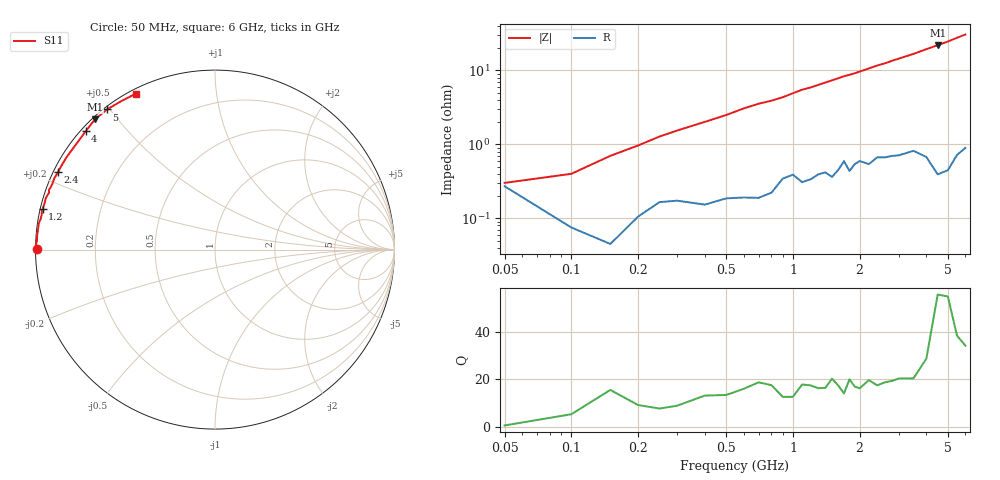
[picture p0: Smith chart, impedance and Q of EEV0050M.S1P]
! Infineon Technologies  Discrete & RF Semiconductors
! BBY55-02W
! Si Tuning Diode in SCD-80
! VR =
! S-Parameters:  June  2000
# GHz  S  MA  R  50
!  f  S11
! GHz  MAG  ANG
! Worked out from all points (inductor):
!   34 points, 50 MHz to 6 GHz, reference 50 ohm
!   read as one part to ground: L = 741 pH near 100 MHz
!   highest Q = 55 at 4.5 GHz (marker M1), where L = 776 pH
!   S11 on the Smith chart (normalised r, x): 50 MHz: 0.01, +0.00; 1.2 GHz: 0.01, +0.12; 2.4 GHz: 0.01, +0.23; 4 GHz: 0.01, +0.39; 5 GHz: 0.01, +0.49; 6 GHz: 0.02, +0.61
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0.05  0.9892 179.7
0.1  0.997 179.1
0.15  0.9982 178.4
0.25  0.9934 177.1
0.5  0.9926 174.3
0.6  0.9924 173.0
0.7  0.9925 171.9
0.8  0.9912 171.1
0.9  0.9864 170.1
1  0.9847 168.8
1.1  0.9879 167.5
1.2  0.9868 166.6
1.4  0.9837 164.4
1.5  0.9859 163.3
1.6  0.9826 162.2
1.7  0.9772 161.1
1.8  0.9832 160.2
1.9  0.9793 159.3
2.2  0.9795 156.0
2.4  0.975 153.8
2.6  0.9752 152.0
3  0.9741 147.8
3.5  0.971 143.0
4  0.9768 137.6
4.5  0.9869 132.6
5  0.9857 127.6
5.5  0.9782 122.1
6  0.9743 117.0
